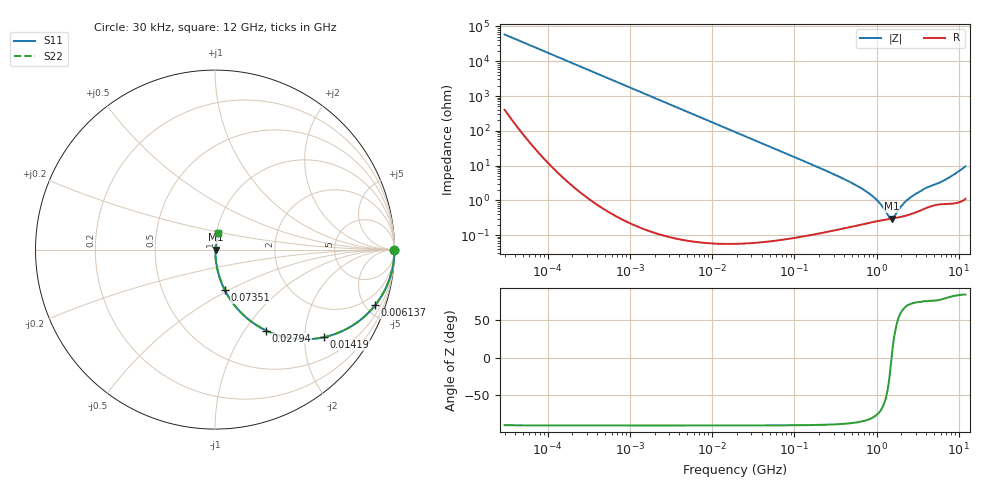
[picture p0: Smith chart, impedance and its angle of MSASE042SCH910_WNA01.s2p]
! MSASE042SCH910_WNA01  S-PARAMETER MODEL  ( General Type )
! Model Generated by TAIYO YUDEN Corporation (http://www.ty-top.com)
! Version 2.0
! TAIYO YUDEN Control No. 131101
! Copyright(c) 2012 TAIYO YUDEN CO.,LTD. All Rights Reserved.
! Product Description (link to TY-COMPAS)
! https://ds.yuden.co.jp/TYCOMPAS/or/detail?pn=MSASE042SCH910JWNA01&u=M
! Products Name : Multilayer Ceramic Capacitors
! Characteristics :
!  Capacitance : 91 pF , Rated Voltage : 16V , TCC : CH / C0H
!  Case Size : 0.4 x 0.2 / 0.016 x 0.008 [mm/inch] , Thickness : 0.2 / 0.008 [mm/inch]
!  (Conditions: Temperature = 25 degC , DC Bias Current/Voltage = 0A / 0V)
! External Node Assignments :
!  1  o---| |---o  2
! GND o---------o GND
! Frequency Range : 0.03MHz  -  12000MHz  [ 401 STEP ]
# MHz S RI R 50
! Freq[MHz].  S11 Real  S11 Imag  S21 Real  S21 Imag  S12 Real  S12 Imag  S22 Real  S22 Imag
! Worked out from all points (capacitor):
!   401 points, 30 kHz to 12 GHz, reference 50 ohm
!   read as one part in series: C = 90.1 pF near 32 kHz
!   lowest |Z| = 298 mohm at 1.524 GHz (marker M1)
!   series resonance near 1.522 GHz, so ESL is about 120 pH
!   S11 on the Smith chart (normalised r, x): 30 kHz: open; 6.137 MHz: 1.00, -5.76; 14.19 MHz: 1.00, -2.49; 27.94 MHz: 1.00, -1.26; 73.51 MHz: 1.00, -0.48; 12 GHz: 1.02, +0.19
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0.03  1 -0.0017  1.45e-05 0.0017  1.45e-05 0.0017  1 -0.0017
0.260295  0.9998 -0.0147  0.00022 0.0147  0.00022 0.0147  0.9998 -0.0147
2.258455  0.9839 -0.1258  0.0161 0.1258  0.0161 0.1258  0.9839 -0.1258
6.13721  0.8923 -0.3099  0.1077 0.3099  0.1077 0.3099  0.8923 -0.3099
9.333359  0.7817 -0.4129  0.2183 0.4129  0.2183 0.4129  0.7817 -0.4129
14.194  0.6076 -0.4881  0.3924 0.4881  0.3924 0.4881  0.6076 -0.4881
18.97367  0.4643 -0.4984  0.5357 0.4984  0.5357 0.4984  0.4643 -0.4984
27.93914  0.2857 -0.4513  0.7143 0.4513  0.7143 0.4513  0.2857 -0.4513
43.88187  0.1397 -0.3459  0.8603 0.3459  0.8603 0.3459  0.1397 -0.3459
73.51358  0.055 -0.2264  0.945 0.2264  0.945 0.2264  0.055 -0.2264
164.6252  0.0121 -0.1047  0.9879 0.1047  0.9879 0.1047  0.0121 -0.1047
433.1624  0.00301 -0.0373  0.997 0.0373  0.997 0.0373  0.00301 -0.0373
749.4426  0.00247 -0.0178  0.9975 0.0178  0.9975 0.0178  0.00247 -0.0178
1068.55  0.00264 -0.00836  0.9974 0.00836  0.9974 0.00836  0.00264 -0.00836
1428.372  0.00289 -0.00149  0.9971 0.00149  0.9971 0.00149  0.00289 -0.00149
1523.532  0.00297 2.61e-05  0.997 -2.61e-05  0.997 -2.61e-05  0.00297 2.61e-05
1625.032  0.00305 0.00149  0.9969 -0.00149  0.9969 -0.00149  0.00305 0.00149
2172.242  0.00357 0.00776  0.9964 -0.00776  0.9964 -0.00776  0.00357 0.00776
2722.352  0.00428 0.0125  0.9957 -0.0125  0.9957 -0.0125  0.00428 0.0125
3881.513  0.00624 0.0209  0.9938 -0.0209  0.9938 -0.0209  0.00624 0.0209
6715.658  0.00913 0.0369  0.9909 -0.0369  0.9909 -0.0369  0.00913 0.0369
12000  0.0193 0.0907  0.9807 -0.0907  0.9807 -0.0907  0.0193 0.0907
